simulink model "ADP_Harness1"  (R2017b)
settings: Solver=FixedStepDiscrete  StartTime=0.0  StopTime=2  FixedStep=0.01  RelTol=1e-3  EnableMultiTasking=on
undefined symbols (not defined in the file): sigbuilder_block
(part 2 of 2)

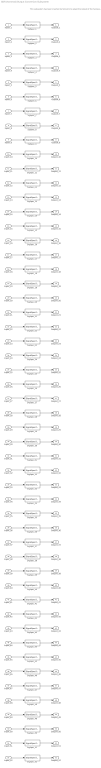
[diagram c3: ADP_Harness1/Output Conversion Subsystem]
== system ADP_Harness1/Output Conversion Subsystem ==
  note: This subsystem has been inserted by Simulink to adapt the output of the harnessed component to the interface required by the sink blocks. Modifying the contents of this subsystem may result in compilation and simulation failure.
  Inport_1 : Inport
  Inport_2 : Inport  Port=2
  Inport_3 : Inport  Port=3
  Inport_4 : Inport  Port=4
  Inport_5 : Inport  Port=5
  Inport_6 : Inport  Port=6
  Inport_7 : Inport  Port=7
  Inport_8 : Inport  Port=8
  Inport_9 : Inport  Port=9
  Inport_10 : Inport  Port=10
  Inport_11 : Inport  Port=11
  Inport_12 : Inport  Port=12
  Inport_13 : Inport  Port=13
  Inport_14 : Inport  Port=14
  Inport_15 : Inport  Port=15
  Inport_16 : Inport  Port=16
  Inport_17 : Inport  Port=17
  Inport_18 : Inport  Port=18
  Inport_19 : Inport  Port=19
  Inport_20 : Inport  Port=20
  Inport_21 : Inport  Port=21
  Inport_22 : Inport  Port=22
  Inport_23 : Inport  Port=23
  Inport_24 : Inport  Port=24
  Inport_25 : Inport  Port=25
  Inport_26 : Inport  Port=26
  Inport_27 : Inport  Port=27
  Inport_28 : Inport  Port=28
  Inport_29 : Inport  Port=29
  Inport_30 : Inport  Port=30
  Inport_31 : Inport  Port=31
  Inport_32 : Inport  Port=32
  Inport_33 : Inport  Port=33
  Inport_34 : Inport  Port=34
  Inport_35 : Inport  Port=35
  Inport_36 : Inport  Port=36
  Inport_37 : Inport  Port=37
  Inport_38 : Inport  Port=38
  Inport_39 : Inport  Port=39
  Inport_40 : Inport  Port=40
  Inport_41 : Inport  Port=41
  Inport_42 : Inport  Port=42
  Inport_43 : Inport  Port=43
  Inport_44 : Inport  Port=44
  Inport_45 : Inport  Port=45
  Inport_46 : Inport  Port=46
  Inport_47 : Inport  Port=47
  Inport_48 : Inport  Port=48
  Inport_49 : Inport  Port=49
  Inport_50 : Inport  Port=50
  Inport_51 : Inport  Port=51
  Inport_52 : Inport  Port=52
  SigSpec_1 : SignalSpecification  OutDataTypeStr=single  Unit=Km/h  Dimensions=[1]  SampleTime=0.01
  SigSpec_{7..14,45,51..52} (11 alike) : SignalSpecification  OutDataTypeStr=uint8  Unit=numb  Dimensions=[1]  SampleTime=0.01
  SigSpec_15 : SignalSpecification  OutDataTypeStr=uint8  Unit=enum  Dimensions=[1]  SampleTime=0.01
  SigSpec_{2..3,6,16,19..21,28..43} (23 alike) : SignalSpecification  OutDataTypeStr=boolean  Unit=flg  Dimensions=[1]  SampleTime=0.01
  SigSpec_17 : SignalSpecification  OutDataTypeStr=single  Unit=W  Dimensions=[1]  SampleTime=0.01
  SigSpec_18 : SignalSpecification  OutDataTypeStr=single  Unit=W  Dimensions=[1]  SampleTime=0.01
  SigSpec_22 : SignalSpecification  OutDataTypeStr=uint16  Unit=Yr  Dimensions=[1]  SampleTime=0.01
  SigSpec_23 : SignalSpecification  OutDataTypeStr=uint8  Unit=Min  Dimensions=[1]  SampleTime=0.01
  SigSpec_24 : SignalSpecification  OutDataTypeStr=uint8  Unit=Day  Dimensions=[1]  SampleTime=0.01
  SigSpec_25 : SignalSpecification  OutDataTypeStr=uint8  Unit=Hour  Dimensions=[1]  SampleTime=0.01
  SigSpec_26 : SignalSpecification  OutDataTypeStr=uint8  Unit=Min  Dimensions=[1]  SampleTime=0.01
  SigSpec_27 : SignalSpecification  OutDataTypeStr=uint8  Unit=S  Dimensions=[1]  SampleTime=0.01
  SigSpec_4 : SignalSpecification  OutDataTypeStr=single  Unit=℃  Dimensions=[1]  SampleTime=0.01
  SigSpec_44 : SignalSpecification  OutDataTypeStr=boolean  Unit=flag  Dimensions=[1]  SampleTime=0.01
  SigSpec_46 : SignalSpecification  OutDataTypeStr=single  Unit=mA  Dimensions=[1]  SampleTime=0.01
  SigSpec_47 : SignalSpecification  OutDataTypeStr=boolean  Unit=flag  Dimensions=[1]  SampleTime=0.01
  SigSpec_48 : SignalSpecification  OutDataTypeStr=uint8  Unit=%  Dimensions=[1]  SampleTime=0.01
  SigSpec_49 : SignalSpecification  OutDataTypeStr=single  Unit=min  Dimensions=[1]  SampleTime=0.01
  SigSpec_5 : SignalSpecification  OutDataTypeStr=single  Unit=numb  Dimensions=[1]  SampleTime=0.01
  SigSpec_50 : SignalSpecification  OutDataTypeStr=uint8  Unit=enum  Dimensions=[1]  SampleTime=0.01
  Outport_1 : Outport
  Outport_2 : Outport  Port=2
  Outport_3 : Outport  Port=3
  Outport_4 : Outport  Port=4
  Outport_5 : Outport  Port=5
  Outport_6 : Outport  Port=6
  Outport_7 : Outport  Port=7
  Outport_8 : Outport  Port=8
  Outport_9 : Outport  Port=9
  Outport_10 : Outport  Port=10
  Outport_11 : Outport  Port=11
  Outport_12 : Outport  Port=12
  Outport_13 : Outport  Port=13
  Outport_14 : Outport  Port=14
  Outport_15 : Outport  Port=15
  Outport_16 : Outport  Port=16
  Outport_17 : Outport  Port=17
  Outport_18 : Outport  Port=18
  Outport_19 : Outport  Port=19
  Outport_20 : Outport  Port=20
  Outport_21 : Outport  Port=21
  Outport_22 : Outport  Port=22
  Outport_23 : Outport  Port=23
  Outport_24 : Outport  Port=24
  Outport_25 : Outport  Port=25
  Outport_26 : Outport  Port=26
  Outport_27 : Outport  Port=27
  Outport_28 : Outport  Port=28
  Outport_29 : Outport  Port=29
  Outport_30 : Outport  Port=30
  Outport_31 : Outport  Port=31
  Outport_32 : Outport  Port=32
  Outport_33 : Outport  Port=33
  Outport_34 : Outport  Port=34
  Outport_35 : Outport  Port=35
  Outport_36 : Outport  Port=36
  Outport_37 : Outport  Port=37
  Outport_38 : Outport  Port=38
  Outport_39 : Outport  Port=39
  Outport_40 : Outport  Port=40
  Outport_41 : Outport  Port=41
  Outport_42 : Outport  Port=42
  Outport_43 : Outport  Port=43
  Outport_44 : Outport  Port=44
  Outport_45 : Outport  Port=45
  Outport_46 : Outport  Port=46
  Outport_47 : Outport  Port=47
  Outport_48 : Outport  Port=48
  Outport_49 : Outport  Port=49
  Outport_50 : Outport  Port=50
  Outport_51 : Outport  Port=51
  Outport_52 : Outport  Port=52
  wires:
  Inport_1/1 -> SigSpec_1/1
  SigSpec_1/1 -> Outport_1/1
  Inport_2/1 -> SigSpec_2/1
  SigSpec_2/1 -> Outport_2/1
  Inport_3/1 -> SigSpec_3/1
  SigSpec_3/1 -> Outport_3/1
  Inport_4/1 -> SigSpec_4/1
  SigSpec_4/1 -> Outport_4/1
  Inport_5/1 -> SigSpec_5/1
  SigSpec_5/1 -> Outport_5/1
  Inport_6/1 -> SigSpec_6/1
  SigSpec_6/1 -> Outport_6/1
  Inport_7/1 -> SigSpec_7/1
  SigSpec_7/1 -> Outport_7/1
  Inport_8/1 -> SigSpec_8/1
  SigSpec_8/1 -> Outport_8/1
  Inport_9/1 -> SigSpec_9/1
  SigSpec_9/1 -> Outport_9/1
  Inport_10/1 -> SigSpec_10/1
  SigSpec_10/1 -> Outport_10/1
  Inport_11/1 -> SigSpec_11/1
  SigSpec_11/1 -> Outport_11/1
  Inport_12/1 -> SigSpec_12/1
  SigSpec_12/1 -> Outport_12/1
  Inport_13/1 -> SigSpec_13/1
  SigSpec_13/1 -> Outport_13/1
  Inport_14/1 -> SigSpec_14/1
  SigSpec_14/1 -> Outport_14/1
  Inport_15/1 -> SigSpec_15/1
  SigSpec_15/1 -> Outport_15/1
  Inport_16/1 -> SigSpec_16/1
  SigSpec_16/1 -> Outport_16/1
  Inport_17/1 -> SigSpec_17/1
  SigSpec_17/1 -> Outport_17/1
  Inport_18/1 -> SigSpec_18/1
  SigSpec_18/1 -> Outport_18/1
  Inport_19/1 -> SigSpec_19/1
  SigSpec_19/1 -> Outport_19/1
  Inport_20/1 -> SigSpec_20/1
  SigSpec_20/1 -> Outport_20/1
  Inport_21/1 -> SigSpec_21/1
  SigSpec_21/1 -> Outport_21/1
  Inport_22/1 -> SigSpec_22/1
  SigSpec_22/1 -> Outport_22/1
  Inport_23/1 -> SigSpec_23/1
  SigSpec_23/1 -> Outport_23/1
  Inport_24/1 -> SigSpec_24/1
  SigSpec_24/1 -> Outport_24/1
  Inport_25/1 -> SigSpec_25/1
  SigSpec_25/1 -> Outport_25/1
  Inport_26/1 -> SigSpec_26/1
  SigSpec_26/1 -> Outport_26/1
  Inport_27/1 -> SigSpec_27/1
  SigSpec_27/1 -> Outport_27/1
  Inport_28/1 -> SigSpec_28/1
  SigSpec_28/1 -> Outport_28/1
  Inport_29/1 -> SigSpec_29/1
  SigSpec_29/1 -> Outport_29/1
  Inport_30/1 -> SigSpec_30/1
  SigSpec_30/1 -> Outport_30/1
  Inport_31/1 -> SigSpec_31/1
  SigSpec_31/1 -> Outport_31/1
  Inport_32/1 -> SigSpec_32/1
  SigSpec_32/1 -> Outport_32/1
  Inport_33/1 -> SigSpec_33/1
  SigSpec_33/1 -> Outport_33/1
  Inport_34/1 -> SigSpec_34/1
  SigSpec_34/1 -> Outport_34/1
  Inport_35/1 -> SigSpec_35/1
  SigSpec_35/1 -> Outport_35/1
  Inport_36/1 -> SigSpec_36/1
  SigSpec_36/1 -> Outport_36/1
  Inport_37/1 -> SigSpec_37/1
  SigSpec_37/1 -> Outport_37/1
  Inport_38/1 -> SigSpec_38/1
  SigSpec_38/1 -> Outport_38/1
  Inport_39/1 -> SigSpec_39/1
  SigSpec_39/1 -> Outport_39/1
  Inport_40/1 -> SigSpec_40/1
  SigSpec_40/1 -> Outport_40/1
  Inport_41/1 -> SigSpec_41/1
  SigSpec_41/1 -> Outport_41/1
  Inport_42/1 -> SigSpec_42/1
  SigSpec_42/1 -> Outport_42/1
  Inport_43/1 -> SigSpec_43/1
  SigSpec_43/1 -> Outport_43/1
  Inport_44/1 -> SigSpec_44/1
  SigSpec_44/1 -> Outport_44/1
  Inport_45/1 -> SigSpec_45/1
  SigSpec_45/1 -> Outport_45/1
  Inport_46/1 -> SigSpec_46/1
  SigSpec_46/1 -> Outport_46/1
  Inport_47/1 -> SigSpec_47/1
  SigSpec_47/1 -> Outport_47/1
  Inport_48/1 -> SigSpec_48/1
  SigSpec_48/1 -> Outport_48/1
  Inport_49/1 -> SigSpec_49/1
  SigSpec_49/1 -> Outport_49/1
  Inport_50/1 -> SigSpec_50/1
  SigSpec_50/1 -> Outport_50/1
  Inport_51/1 -> SigSpec_51/1
  SigSpec_51/1 -> Outport_51/1
  Inport_52/1 -> SigSpec_52/1
  SigSpec_52/1 -> Outport_52/1
